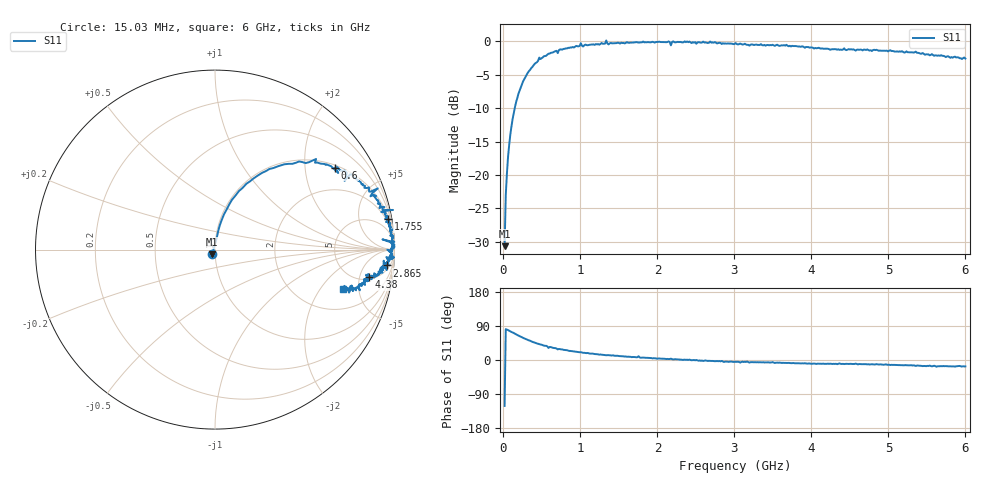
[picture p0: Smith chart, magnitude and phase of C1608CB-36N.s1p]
!	Network	Analyzer	HP8753E.07.74:	Oct	30	2002	Serial	No.	JP38451487
!	Hewlett-Packard
!	28	Aug	2009	8:09:20
!	Frequency	S11
#	HZ	S	RI	R	50
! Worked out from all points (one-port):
!   400 points, 15.03 MHz to 6 GHz, reference 50 ohm
!   lowest |S11| = -30.6 dB at 15.03 MHz (marker M1), VSWR 1.06, Z = 48.4 - j2.43 ohm
!   |S11| at or under -10 dB: start of sweep to 146.6 MHz
!   S11 on the Smith chart (normalised r, x): 15.03 MHz: 0.97, -0.05; 600 MHz: 1.08, +2.87; 1.755 GHz: 1, +11; 2.865 GHz: 8, -18; 4.38 GHz: 5.57, -6.93; 6 GHz: 3.43, -3.32
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1.502992e7  -0.0152 -0.0251
3.002985e7  0.0106 0.0697
6.00297e7  0.0264 0.135
1.050295e8  0.0652 0.224
1.650292e8  0.133 0.326
3.450283e8  0.385 0.475
4.650277e8  0.563 0.505
6.00027e8  0.669 0.457
7.650262e8  0.768 0.406
1.005025e9  0.907 0.341
1.320023e9  0.937 0.22
1.335023e9  0.992 0.221
1.365023e9  0.926 0.21
1.515022e9  0.948 0.171
1.725021e9  0.981 0.124
1.755021e9  0.966 0.171
1.785021e9  0.978 0.1
2.145019e9  0.999 0.0429
2.175019e9  0.933 0.057
2.205019e9  1 0.026
2.265019e9  0.992 0.0287
2.865016e9  0.958 -0.0884
3.015015e9  0.968 -0.0822
3.765011e9  0.914 -0.127
4.380008e9  0.856 -0.152
4.515007e9  0.86 -0.153
5.265004e9  0.805 -0.201
6e9  0.711 -0.217
